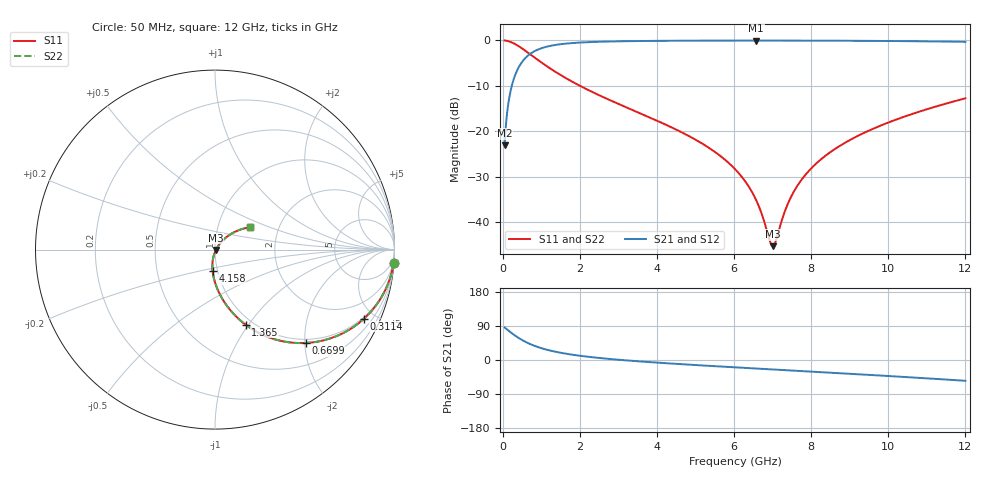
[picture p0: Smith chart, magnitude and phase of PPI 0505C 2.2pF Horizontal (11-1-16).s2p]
# MHz S MA R 50
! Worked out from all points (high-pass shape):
!   1601 points, 50 MHz to 12 GHz, reference 50 ohm
!   highest |S21| = -0.05 dB at 6.578 GHz (marker M1); lowest = -23.1 dB at 50 MHz (marker M2)
!   |S21| within 3 dB of the highest: 700.6 MHz to end of sweep
!   lowest |S11| = -45.3 dB at 7.003 GHz (marker M3), VSWR 1.01, Z = 50.5 - j0.249 ohm
!   |S11| at or under -10 dB: 2.003 GHz to end of sweep
!   |S22| runs from -45.3 to 0.0 dB; largest |S21 - S12| = 0
!   S11 on the Smith chart (normalised r, x): 50 MHz: 1, -27; 311.4 MHz: 0.92, -4.36; 669.9 MHz: 0.92, -2.02; 1.365 GHz: 0.92, -0.97; 4.158 GHz: 0.95, -0.23; 12 GHz: 1.42, +0.38
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50  0.9975 -4.2  0.0702 85.8  0.0702 85.8  0.9975 -4.2
169.5  0.9726 -14.0  0.2321 75.9  0.2321 75.9  0.9726 -14.0
311.4062  0.9155 -24.8  0.4018 65.1  0.4018 65.1  0.9155 -24.8
475.7188  0.8297 -35.6  0.5573 54.3  0.5573 54.3  0.8297 -35.6
669.9062  0.7248 -45.9  0.6877 44.0  0.6877 44.0  0.7248 -45.9
991.0625  0.5765 -58.2  0.8153 31.6  0.8153 31.6  0.5765 -58.2
1364.5  0.4514 -67.8  0.8902 21.9  0.8902 21.9  0.4514 -67.8
2044.156  0.3097 -78.9  0.9481 10.6  0.9481 10.6  0.3097 -78.9
4038.312  0.1286 -95.5  0.9876 -7.2  0.9876 -7.2  0.1286 -95.5
4157.812  0.122 -96.2  0.9884 -8.0  0.9884 -8.0  0.122 -96.2
5278.125  0.0687 -101.3  0.9929 -15.0  0.9929 -15.0  0.0687 -101.3
6025  0.03834 -102.1  0.994 -19.4  0.994 -19.4  0.03834 -102.1
6577.688  0.01733 -95.1  0.9943 -22.5  0.9943 -22.5  0.01733 -95.1
6928.719  0.006197 -54.1  0.9942 -24.5  0.9942 -24.5  0.006197 -54.1
7003.406  0.005437 -27.0  0.9941 -24.9  0.9941 -24.9  0.005437 -27.0
7078.094  0.006094 0.6  0.9941 -25.4  0.9941 -25.4  0.006094 0.6
7302.156  0.0126 36.9  0.9939 -26.6  0.9939 -26.6  0.0126 36.9
7488.875  0.01936 45.1  0.9936 -27.7  0.9936 -27.7  0.01936 45.1
8019.156  0.03972 50.5  0.9927 -30.7  0.9927 -30.7  0.03972 50.5
8833.25  0.07277 49.4  0.9902 -35.3  0.9902 -35.3  0.07277 49.4
10013.31  0.1253 44.3  0.984 -42.3  0.984 -42.3  0.1253 44.3
12000  0.2304 32.8  0.963 -54.8  0.963 -54.8  0.2304 32.8
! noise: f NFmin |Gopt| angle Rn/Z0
50  0.0007263  0.9421  2.075  0.002804
1372  0.005657  0.7599  6.074  0.00476
2701  0.009237  0.7175  10.52  0.006414
4031  0.01247  0.6938  15.03  0.007812
5360  0.0156  0.6795  19.51  0.009149
6682  0.01871  0.6717  23.89  0.01052
8012  0.02194  0.6689  28.21  0.01201
9341  0.02536  0.6703  32.42  0.01369
1.067e+04  0.02906  0.6755  36.53  0.01564
1.2e+04  0.03314  0.6839  40.53  0.01798
